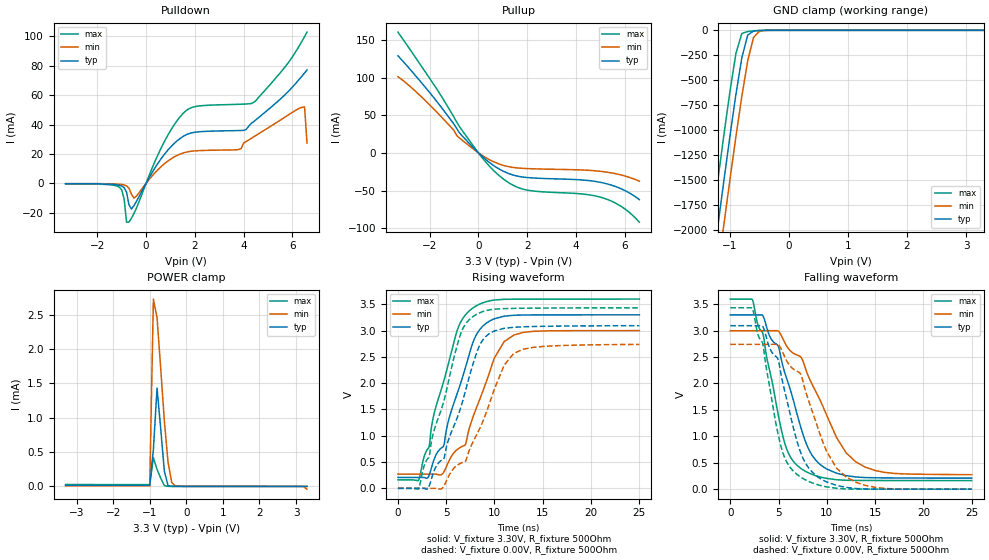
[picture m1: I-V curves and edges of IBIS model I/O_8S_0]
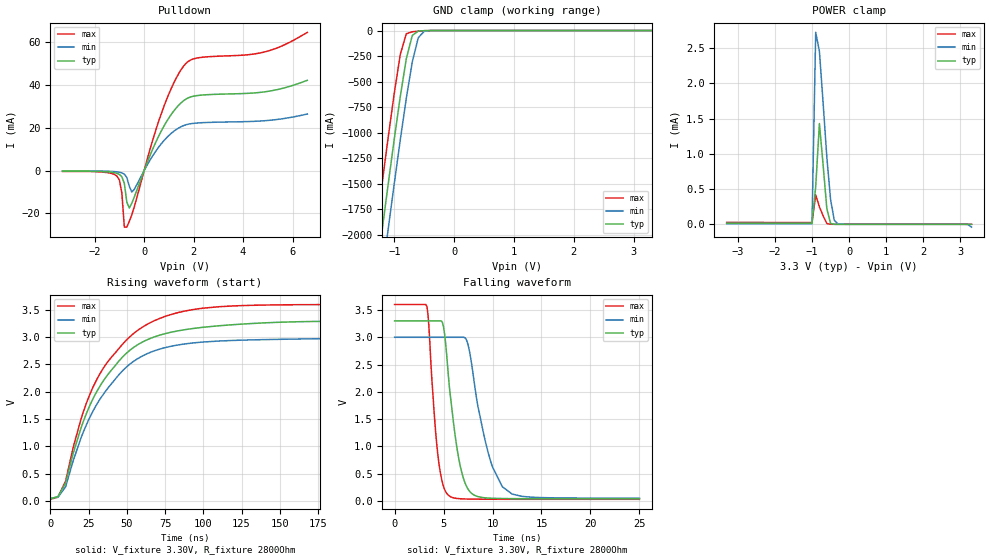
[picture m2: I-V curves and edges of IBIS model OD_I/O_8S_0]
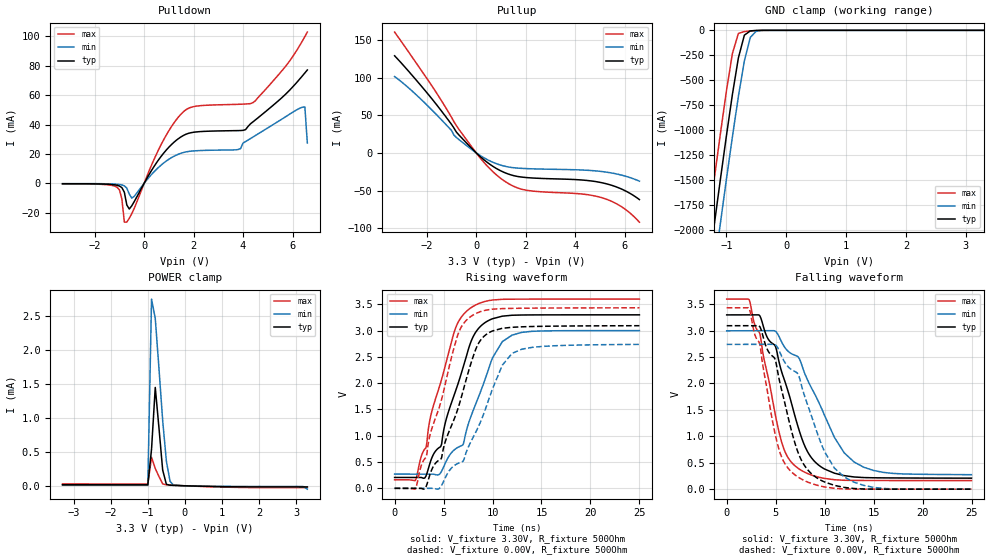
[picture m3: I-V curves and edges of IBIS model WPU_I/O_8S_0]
[IBIS Ver]   3.2
[File Name]   lm3s2651_lqfp_v0p1.ibs
[File Rev]   0.1
[Date]   02/19/2010
[Source]   From silicon level SPICE simulations at Texas Instruments
[Notes]   Initial Release of IBIS model
   LM3S2651, Revision A2, 100 LQFP
[Disclaimer] Texas Instruments Confidential - Advance Product Information
   < Software License Agreement >
  Texas Instruments (TI) is supplying this software for use solely and
  exclusively on TI's Stellaris Family of microcontroller products.
  The software is owned by TI and/or its suppliers, and is protected under
  applicable copyright laws.  All rights are reserved.  Any use in violation
  of the foregoing restrictions may subject the user to criminal sanctions
  under applicable laws, as well as to civil liability for the breach of the
  terms and conditions of this license.
  THIS SOFTWARE IS PROVIDED "AS IS".  NO WARRANTIES, WHETHER EXPRESS, IMPLIED
  OR STATUTORY, INCLUDING, BUT NOT LIMITED TO, IMPLIED WARRANTIES OF
  MERCHANTABILITY AND FITNESS FOR A PARTICULAR PURPOSE APPLY TO THIS SOFTWARE.
  LMI SHALL NOT, IN ANY CIRCUMSTANCES, BE LIABLE FOR SPECIAL, INCIDENTAL, OR
  CONSEQUENTIAL DAMAGES, FOR ANY REASON WHATSOEVER.
[Copyright]   Copyright (c) 2010 Texas Instruments.  All rights reserved.
[Component]   LM3S2651 100LQFP
[Manufacturer]  Texas Instruments
[Package]
| 100-pin LQFP
| variable   typ   min   max
R_pkg   125.000m   98.000m   152.000m
L_pkg   7.745nH   6.720nH   8.770nH
C_pkg   0.745pF   0.660pF   0.830pF
[Pin]  signal_name   model_name
   1   ADC0   NC
   2   ADC1   NC
   3   VDDA   POWER
   4   GNDA   GND
   5   ADC2   NC
   6   ADC3   NC
   7   LDO   POWER
   8   VDD   POWER
   9   GND   GND
  10   PD0_CAN0Rx   ProgBuff1
  11   PD1_CAN0Tx   ProgBuff1
  12   PD2_U1Rx   ProgBuff1
  13   PD3_U1Tx   ProgBuff1
  14   VDD25   POWER
  15   GND   GND
  16   PG3   ProgBuff2
  17   PG2   ProgBuff2
  18   PG1_U2Tx   ProgBuff1
  19   PG0_U2Rx   ProgBuff1
  20   VDD   POWER
  21   GND   GND
  22   NC   NC
  23   PC6_CCP3   ProgBuff1
  24   PC5_C0o   ProgBuff1
  25   PC4   ProgBuff1
  26   PA0_U0Rx   ProgBuff1
  27   PA1_U0Tx   ProgBuff1
  28   PA2_SSI0Clk   ProgBuff1
  29   PA3_SSI0Fss   ProgBuff1
  30   PA4_SSI0Rx   ProgBuff1
  31   PA5_SSI0Tx   ProgBuff1
  32   VDD   POWER
  33   GND   GND
  34   PA6_CCP1   ProgBuff1
  35   PA7_CCP4   ProgBuff1
  36   PG7   ProgBuff2
  37   PG6   ProgBuff2
  38   VDD25   POWER
  39   GND   GND
  40   PG5   ProgBuff2
  41   PG4   ProgBuff2
  42   PF7   ProgBuff2
  43   PF6   ProgBuff2
  44   VDD   POWER
  45   GND   GND
  46   PF5   ProgBuff2
  47   PF0_PWM0   ProgBuff1
  48   OSC0   NC
  49   OSC1   NC
  50   WAKE   NC
  51   HIB   NC
  52   XOSC0   NC
  53   XOSC1   NC
  54   GND   GND
  55   VBAT   POWER
  56   VDD   POWER
  57   GND   GND
  58   PF4   ProgBuff1
  59   PF3   ProgBuff1
  60   PF2   ProgBuff1
  61   PF1_PWM1   ProgBuff1
  62   VDD25   POWER
  63   GND   GND
  64   RST   NC
  65   CMOD0   NC
  66   PB0_CCP0   ProgBuff1
  67   PB1_CCP2   ProgBuff1
  68   VDD   POWER
  69   GND   GND
  70   PB2_I2C0SCL   ProgBuff1
  71   PB3_I2C0SDA   ProgBuff1
  72   PE0_SSI1Clk   ProgBuff1
  73   PE1_SSI1Fss   ProgBuff1
  74   PE2_SSI1Rx   ProgBuff1
  75   PE3_SSI1Tx   ProgBuff1
  76   CMOD1   NC
  77   PC3_TDO_SWO   ProgBuff1
  78   PC2_TDI   ProgBuff1
  79   PC1_TMS_SWDIO   ProgBuff1
  80   PC0_TCK_SWCLK   ProgBuff1
  81   VDD   POWER
  82   GND   GND
  83   NC   NC
  84   NC   NC
  85   PH1_PWM3   ProgBuff2
  86   PH0_PWM2   ProgBuff2
  87   GND   GND
  88   VDD25   POWER
  89   PB7_TRST   ProgBuff1
  90   PB6   ProgBuff1
  91   PB5_CCP5   ProgBuff1
  92   PB4   ProgBuff1
  93   VDD   POWER
  94   GND   GND
  95   PD4   ProgBuff0
  96   PD5   ProgBuff0
  97   GNDA   GND
  98   VDDA   POWER
  99   PD6_Fault   ProgBuff0
 100   PD7   ProgBuff0
[Model Selector]   ProgBuff0
I/O_2_0   2 mA buffer without slew rate control
I/O_4_0   4 mA buffer without slew rate control
I/O_8_0   8 mA buffer without slew rate control
I/O_8S_0   8 mA buffer with slew rate control
OD_I/O_2_0   open-drain 2 mA buffer without slew rate control
OD_I/O_4_0   open-drain 4 mA buffer without slew rate control
OD_I/O_8_0   open-drain 8 mA buffer without slew rate control
OD_I/O_8S_0   open-drain 8 mA buffer with slew rate control
WPU_I/O_2_0   weak pullup 2 mA buffer without slew rate control
WPU_I/O_4_0   weak pullup 4 mA buffer without slew rate control
WPU_I/O_8_0   weak pullup 8 mA buffer without slew rate control
WPU_I/O_8S_0   weak pullup 8 mA buffer with slew rate control
WPD_I/O_2_0   weak pulldown 2 mA buffer without slew rate control
WPD_I/O_4_0   weak pulldown 4 mA buffer without slew rate control
WPD_I/O_8_0   weak pulldown 8 mA buffer without slew rate control
WPD_I/O_8S_0   weak pulldown 8 mA buffer with slew rate control
[Model Selector]   ProgBuff1
I/O_2_1   2 mA buffer without slew rate control
I/O_4_1   4 mA buffer without slew rate control
I/O_8_1   8 mA buffer without slew rate control
I/O_8S_1   8 mA buffer with slew rate control
OD_I/O_2_1   open-drain 2 mA buffer without slew rate control
OD_I/O_4_1   open-drain 4 mA buffer without slew rate control
OD_I/O_8_1   open-drain 8 mA buffer without slew rate control
OD_I/O_8S_1   open-drain 8 mA buffer with slew rate control
WPU_I/O_2_1   weak pullup 2 mA buffer without slew rate control
WPU_I/O_4_1   weak pullup 4 mA buffer without slew rate control
WPU_I/O_8_1   weak pullup 8 mA buffer without slew rate control
WPU_I/O_8S_1   weak pullup 8 mA buffer with slew rate control
WPD_I/O_2_1   weak pulldown 2 mA buffer without slew rate control
WPD_I/O_4_1   weak pulldown 4 mA buffer without slew rate control
WPD_I/O_8_1   weak pulldown 8 mA buffer without slew rate control
WPD_I/O_8S_1   weak pulldown 8 mA buffer with slew rate control
[Model Selector]   ProgBuff2
I/O_2_2   2 mA buffer without slew rate control
I/O_4_2   4 mA buffer without slew rate control
I/O_8_2   8 mA buffer without slew rate control
I/O_8S_2   8 mA buffer with slew rate control
OD_I/O_2_2   open-drain 2 mA buffer without slew rate control
OD_I/O_4_2   open-drain 4 mA buffer without slew rate control
OD_I/O_8_2   open-drain 8 mA buffer without slew rate control
OD_I/O_8S_2   open-drain 8 mA buffer with slew rate control
WPU_I/O_2_2   weak pullup 2 mA buffer without slew rate control
WPU_I/O_4_2   weak pullup 4 mA buffer without slew rate control
WPU_I/O_8_2   weak pullup 8 mA buffer without slew rate control
WPU_I/O_8S_2   weak pullup 8 mA buffer with slew rate control
WPD_I/O_2_2   weak pulldown 2 mA buffer without slew rate control
WPD_I/O_4_2   weak pulldown 4 mA buffer without slew rate control
WPD_I/O_8_2   weak pulldown 8 mA buffer without slew rate control
WPD_I/O_8S_2   weak pulldown 8 mA buffer with slew rate control
| Models and submodels in the file (48): I/O_2_0 (I/O), I/O_4_0 (I/O), I/O_8_0 (I/O), I/O_8S_0 (I/O), OD_I/O_2_0 (I/O_open_drain), OD_I/O_4_0 (I/O_open_drain), OD_I/O_8_0 (I/O_open_drain), OD_I/O_8S_0 (I/O_open_drain), WPU_I/O_2_0 (I/O), WPU_I/O_4_0 (I/O), WPU_I/O_8_0 (I/O), WPU_I/O_8S_0 (I/O), WPD_I/O_2_0 (I/O), WPD_I/O_4_0 (I/O), WPD_I/O_8_0 (I/O), WPD_I/O_8S_0 (I/O), I/O_2_1 (I/O), I/O_4_1 (I/O), I/O_8_1 (I/O), I/O_8S_1 (I/O), OD_I/O_2_1 (I/O_open_drain), OD_I/O_4_1 (I/O_open_drain), OD_I/O_8_1 (I/O_open_drain), OD_I/O_8S_1 (I/O_open_drain), WPU_I/O_2_1 (I/O), WPU_I/O_4_1 (I/O), WPU_I/O_8_1 (I/O), WPU_I/O_8S_1 (I/O), WPD_I/O_2_1 (I/O), WPD_I/O_4_1 (I/O), WPD_I/O_8_1 (I/O), WPD_I/O_8S_1 (I/O), I/O_2_2 (I/O), I/O_4_2 (I/O), I/O_8_2 (I/O), I/O_8S_2 (I/O), OD_I/O_2_2 (I/O_open_drain), OD_I/O_4_2 (I/O_open_drain), OD_I/O_8_2 (I/O_open_drain), OD_I/O_8S_2 (I/O_open_drain), WPU_I/O_2_2 (I/O), WPU_I/O_4_2 (I/O), WPU_I/O_8_2 (I/O), WPU_I/O_8S_2 (I/O), WPD_I/O_2_2 (I/O), WPD_I/O_4_2 (I/O), WPD_I/O_8_2 (I/O), WPD_I/O_8S_2 (I/O)
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[Model]   I/O_8S_0
Model_type   I/O
Vinl = 1.26
Vinh = 2.04
Vmeas = 1.65
| variable   typ   min   max
C_comp   9.739pF   9.739pF   9.739pF
[Model Spec]
Vinh+   1.91   1.78   2.04
Vinh-   1.90   1.76   2.03
Vinl+   1.40   1.27   1.54
Vinl-   1.39   1.26   1.53
| variable   typ   min   max
[Temperature Range]  25   85   -40
[Voltage Range]   3.3V   3.0V   3.6V
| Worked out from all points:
|   slope of the pulldown table from 0 to 0.495 V, typ, clamps not added: 35.8 ohm
|   slope of the pullup table from 0 to 0.495 V, typ, clamps not added: 35.8 ohm
|   GND clamp passes 1 mA (typ) near -0.48 V on its own axis
|   POWER clamp passes 1 mA (typ) near -0.73 V on its own axis
|   falling waveform, V_fixture 3.30V, R_fixture 500Ohm: 20-80 % time 2.93ns typ, 4.09ns min, 2.25ns max; typ from 3.3 V to 0.208 V
|   rising waveform, V_fixture 3.30V, R_fixture 500Ohm: 20-80 % time 2.83ns typ, 3.04ns min, 2.71ns max; typ from 0.208 V to 3.3 V
|   falling waveform, V_fixture 0.00V, R_fixture 500Ohm: 20-80 % time 2.55ns typ, 3.29ns min, 2.08ns max; typ from 3.09 V to 0 V
|   rising waveform, V_fixture 0.00V, R_fixture 500Ohm: 20-80 % time 3.13ns typ, 3.58ns min, 2.86ns max; typ from 0 V to 3.09 V
[Pulldown]
|  Voltage   I(typ)   I(min)   I(max)
-3.3V     -256.6uA   -145.6uA   -364.5uA
-1.1V     -1.273mA   -587.5uA   -2.567mA
-900mV    -2.885mA   -1.061mA   -10.54mA
-800mV    -5.993mA   -1.67mA    -26.39mA
-700mV    -14.71mA   -3.215mA   -26.33mA
-500mV    -15.26mA   -10mA      -20.66mA
600mV     16.36mA    11.13mA    23.41mA
1.5V      31.68mA    20.52mA    47.2mA
3.8V      35.88mA    22.99mA    53.74mA
4.4V      41.81mA    31.48mA    54.89mA
6.5V      75.06mA    51.95mA    99.78mA
6.6V      77.08mA    27.42mA    102.8mA
[Pullup]
|  Voltage   I(typ)   I(min)   I(max)
-3.3V     128.9mA    101.3mA    160.4mA
-2V       80.13mA    63.77mA    99.04mA
-1V       37.9mA     29.83mA    47.32mA
-700mV    23.81mA    17.7mA     31.28mA
300mV     -8.845mA   -6.303mA   -12.15mA
1V        -23.99mA   -16.37mA   -34.1mA
1.5V      -30.13mA   -19.7mA    -44.22mA
2V        -32.73mA   -20.87mA   -49.46mA
4.3V      -36.12mA   -22.8mA    -54.75mA
5.1V      -39.81mA   -24.88mA   -59.77mA
5.9V      -48.4mA    -29.75mA   -72.06mA
6.6V      -62.06mA   -37.61mA   -92.08mA
[GND Clamp]
|  Voltage   I(typ)   I(min)   I(max)
-3.3V     -11.72A    -12.12A    -11.3A
-1.4V     -2.845A    -3.285A    -2.387A
-1.3V     -2.39A     -2.831A    -1.93A
-1.2V     -1.938A    -2.38A     -1.478A
-1.1V     -1.494A    -1.934A    -1.036A
-1V       -1.059A    -1.496A    -610.6mA
-900mV    -645mA     -1.069A    -232.9mA
-800mV    -277.1mA   -664.4mA   -31.59mA
-700mV    -48.56mA   -306.6mA   -12.09mA
-600mV    -5.558mA   -70.2mA    -6.272mA
-500mV    -1.167mA   -7.88mA    -2.167mA
3.3V      2.282nA    3.101uA    451.3pA
[POWER Clamp]
|  Voltage   I(typ)   I(min)   I(max)
-3.3V     15.18uA    8.315uA    27.48uA
-1V       14.14uA    7.74uA     25.63uA
-900mV    536uA      2.726mA    416.7uA
-800mV    1.43mA     2.454mA    247.6uA
-700mV    840.7uA    1.719mA    119.9uA
-600mV    221.2uA    951.5uA    11.58uA
-500mV    12.35uA    355.6uA    955.3nA
-400mV    305.2nA    58.59uA    44.3nA
-300mV    9.515nA    3.101uA    1.472nA
3.1V      1.302nA    -112.7nA   143.5pA
3.2V      1.207nA    -2.287uA   131.7pA
3.3V      -104.8pA   -40.34uA   119.2pA
[Ramp]
| variable   typ   min   max
dV/dt_f   1.85/2.93n   1.63/4.09n   2.06/2.25n
dV/dt_r   1.85/3.13n   1.64/3.58n   2.06/2.86n
R_load = 500Ohm
[Falling Waveform]
V_fixture = 3.30V
V_fixture_min = 3.00V
V_fixture_max = 3.60V
R_fixture = 500Ohm
|   Time   V(typ)   V(min)   V(max)
0s        3.298V     2.996V     3.597V
2.3ns     3.298V     2.998V     3.585V
3.4ns     3.276V     2.998V     2.936V
5ns       2.692V     2.987V     1.378V
5.6ns     2.229V     2.79V      898.3mV
7.2ns     1.235V     2.517V     407.7mV
9.1ns     502.1mV    1.761V     241.2mV
11ns      302.3mV    979.8mV    178.8mV
13ns      231mV      515.9mV    165.4mV
25ns      208.4mV    274.1mV    162.4mV
[Rising Waveform]
V_fixture = 3.30V
V_fixture_min = 3.00V
V_fixture_max = 3.60V
R_fixture = 500Ohm
|   Time   V(typ)   V(min)   V(max)
0s        207.7mV    271.2mV    162.2mV
2.1ns     207.5mV    270.5mV    146.6mV
3.2ns     232.7mV    270.2mV    771.4mV
4.8ns     840.9mV    326.1mV    2.073V
6.1ns     1.783V     732.4mV    2.98V
7ns       2.303V     833.1mV    3.299V
7.7ns     2.739V     1.319V     3.42V
10ns      3.225V     2.483V     3.58V
12ns      3.291V     2.913V     3.596V
25ns      3.299V     2.999V     3.598V
[Falling Waveform]
V_fixture = 0.00V
V_fixture_min = 0.00V
V_fixture_max = 0.00V
R_fixture = 500Ohm
|   Time   V(typ)   V(min)   V(max)
0s        3.093V     2.739V     3.433V
2.3ns     3.093V     2.74V      3.421V
3.4ns     3.071V     2.74V      2.73V
4.9ns     2.477V     2.739V     1.087V
5.3ns     2.13V      2.643V     778.7mV
7ns       852.9mV    2.223V     266.6mV
8.1ns     406.7mV    1.685V     148.2mV
10ns      135.5mV    708.4mV    42.72mV
12ns      33.41mV    230.5mV    3.849mV
25ns      39.44uV    90.62uV    23.66uV
[Rising Waveform]
V_fixture = 0.00V
V_fixture_min = 0.00V
V_fixture_max = 0.00V
R_fixture = 500Ohm
|   Time   V(typ)   V(min)   V(max)
0s        402.7uV    2.355mV    175.9uV
2.1ns     186.9uV    995.9uV    -14.86mV
3.1ns     -4.815mV   567.3uV    569mV
4.6ns     543.7mV    4.108mV    1.563V
6.4ns     1.478V     468.1mV    2.886V
7.7ns     2.319V     853mV      3.256V
9.1ns     2.885V     1.418V     3.377V
11ns      3.043V     2.342V     3.417V
12ns      3.062V     2.567V     3.421V
25ns      3.092V     2.736V     3.432V
[Model]   OD_I/O_8S_0
Model_type   I/O_open_drain
Polarity   Inverting
Vinl = 1.26
Vinh = 2.04
Vmeas = 1.65
Rref = 2800
Vref = 3.3
| variable   typ   min   max
C_comp   9.739pF   9.739pF   9.739pF
[Model Spec]
Vinh+   1.91   1.78   2.04
Vinh-   1.90   1.76   2.03
Vinl+   1.40   1.27   1.54
Vinl-   1.39   1.26   1.53
| variable   typ   min   max
[Temperature Range]  25   85   -40
[Voltage Range]   3.3V   3.0V   3.6V
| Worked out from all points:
|   slope of the pulldown table from 0 to 0.495 V, typ, clamps not added: 35.8 ohm
|   GND clamp passes 1 mA (typ) near -0.48 V on its own axis
|   POWER clamp passes 1 mA (typ) near -0.73 V on its own axis
|   falling waveform, V_fixture 3.30V, R_fixture 2800Ohm: 20-80 % time 1.32ns typ, 2.02ns min, 884ps max; typ from 3.3 V to 0.038 V
|   rising waveform, V_fixture 3.30V, R_fixture 2800Ohm: 20-80 % time 34.2ns typ, 34ns min, 34.6ns max; typ from 0.038 V to 3.3 V
[Pulldown]
|  Voltage   I(typ)   I(min)   I(max)
-3.3V     -256.6uA   -145.6uA   -364.5uA
-1.1V     -1.273mA   -587.5uA   -2.567mA
-900mV    -2.885mA   -1.061mA   -10.54mA
-800mV    -5.993mA   -1.67mA    -26.39mA
-700mV    -14.71mA   -3.215mA   -26.33mA
-600mV    -17.43mA   -7.321mA   -23.73mA
-500mV    -15.26mA   -10mA      -20.66mA
700mV     18.62mA    12.61mA    26.75mA
1.2V      27.84mA    18.36mA    40.91mA
1.7V      33.44mA    21.41mA    50.13mA
4.9V      36.8mA     23.3mA     55.47mA
6.6V      42.15mA    26.42mA    64.53mA
[GND Clamp]
|  Voltage   I(typ)   I(min)   I(max)
-3.3V     -11.72A    -12.12A    -11.3A
-1.4V     -2.845A    -3.285A    -2.387A
-1.3V     -2.39A     -2.831A    -1.93A
-1.2V     -1.938A    -2.38A     -1.478A
-1.1V     -1.494A    -1.934A    -1.036A
-1V       -1.059A    -1.496A    -610.6mA
-900mV    -645mA     -1.069A    -232.9mA
-800mV    -277.1mA   -664.4mA   -31.59mA
-700mV    -48.56mA   -306.6mA   -12.09mA
-600mV    -5.558mA   -70.2mA    -6.272mA
-500mV    -1.167mA   -7.88mA    -2.167mA
3.3V      2.282nA    3.101uA    451.3pA
[POWER Clamp]
|  Voltage   I(typ)   I(min)   I(max)
-3.3V     15.18uA    8.315uA    27.48uA
-1V       14.14uA    7.74uA     25.63uA
-900mV    536uA      2.726mA    416.7uA
-800mV    1.43mA     2.454mA    247.6uA
-700mV    840.7uA    1.719mA    119.9uA
-600mV    221.2uA    951.5uA    11.58uA
-500mV    12.35uA    355.6uA    955.3nA
-400mV    305.2nA    58.59uA    44.3nA
-300mV    9.515nA    3.101uA    1.472nA
3.1V      1.302nA    -112.7nA   143.5pA
3.2V      1.207nA    -2.287uA   131.7pA
3.3V      -104.8pA   -40.34uA   119.2pA
[Ramp]
| variable   typ   min   max
dV/dt_f   1.96/1.32n   1.77/2.02n   2.14/0.88n
dV/dt_r   1.96/34.24n   1.77/34.01n   2.14/34.63n
R_load = 2800Ohm
[Falling Waveform]
V_fixture = 3.30V
V_fixture_min = 3.00V
V_fixture_max = 3.60V
R_fixture = 2800Ohm
|   Time   V(typ)   V(min)   V(max)
0s        3.3V       2.999V     3.6V
3.3ns     3.3V       2.999V     3.564V
4.4ns     3.3V       2.999V     872.1mV
5ns       3.186V     2.999V     262.6mV
5.5ns     2.279V     2.999V     103.6mV
6.4ns     934mV      2.999V     44.88mV
7.3ns     283.8mV    2.965V     35.58mV
9.4ns     54.75mV    993.7mV    31.53mV
11ns      44.17mV    261mV      30.69mV
25ns      37.97mV    50.43mV    29.46mV
[Rising Waveform]
V_fixture = 3.30V
V_fixture_min = 3.00V
V_fixture_max = 3.60V
R_fixture = 2800Ohm
|   Time   V(typ)   V(min)   V(max)
0s        38.08mV    50.7mV     29.48mV
5ns       80.81mV    66.81mV    69.32mV
10ns      324.3mV    257.9mV    361.8mV
20ns      1.329V     1.148V     1.491V
32ns      2.082V     1.844V     2.308V
49ns      2.686V     2.433V     2.925V
65ns      2.973V     2.718V     3.261V
85ns      3.124V     2.865V     3.461V
110ns     3.209V     2.93V      3.558V
250ns     3.298V     2.994V     3.599V
[Model]   WPU_I/O_8S_0
Model_type   I/O
Vinl = 1.26
Vinh = 2.04
Vmeas = 1.65
| variable   typ   min   max
C_comp   9.739pF   9.739pF   9.739pF
[Model Spec]
Vinh+   1.91   1.78   2.04
Vinh-   1.90   1.76   2.03
Vinl+   1.40   1.27   1.54
Vinl-   1.39   1.26   1.53
| variable   typ   min   max
[Temperature Range]  25   85   -40
[Voltage Range]   3.3V   3.0V   3.6V
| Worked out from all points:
|   slope of the pulldown table from 0 to 0.495 V, typ, clamps not added: 35.8 ohm
|   slope of the pullup table from 0 to 0.495 V, typ, clamps not added: 35.8 ohm
|   GND clamp passes 1 mA (typ) near -0.48 V on its own axis
|   POWER clamp passes 1 mA (typ) near -0.73 V on its own axis
|   falling waveform, V_fixture 3.30V, R_fixture 500Ohm: 20-80 % time 2.93ns typ, 4.09ns min, 2.25ns max; typ from 3.3 V to 0.208 V
|   rising waveform, V_fixture 3.30V, R_fixture 500Ohm: 20-80 % time 2.83ns typ, 3.04ns min, 2.71ns max; typ from 0.208 V to 3.3 V
|   falling waveform, V_fixture 0.00V, R_fixture 500Ohm: 20-80 % time 2.55ns typ, 3.29ns min, 2.08ns max; typ from 3.09 V to 0 V
|   rising waveform, V_fixture 0.00V, R_fixture 500Ohm: 20-80 % time 3.13ns typ, 3.58ns min, 2.86ns max; typ from 0 V to 3.09 V
[Pulldown]
|  Voltage   I(typ)   I(min)   I(max)
-3.3V     -256.4uA   -145.5uA   -364.3uA
-1.1V     -1.272mA   -586.9uA   -2.565mA
-900mV    -2.884mA   -1.06mA    -10.53mA
-800mV    -5.991mA   -1.669mA   -26.38mA
-700mV    -14.71mA   -3.213mA   -26.31mA
-500mV    -15.24mA   -9.997mA   -20.64mA
600mV     16.38mA    11.14mA    23.43mA
1.5V      31.7mA     20.53mA    47.23mA
3.8V      35.88mA    22.99mA    53.74mA
4.4V      41.81mA    31.48mA    54.88mA
6.5V      75.06mA    51.95mA    99.78mA
6.6V      77.08mA    27.42mA    102.8mA
[Pullup]
|  Voltage   I(typ)   I(min)   I(max)
-3.3V     128.9mA    101.3mA    160.4mA
-2V       80.13mA    63.77mA    99.04mA
-1V       37.9mA     29.83mA    47.32mA
-700mV    23.8mA     17.69mA    31.27mA
300mV     -8.84mA    -6.3mA     -12.15mA
1V        -23.98mA   -16.37mA   -34.08mA
1.5V      -30.12mA   -19.69mA   -44.19mA
2V        -32.71mA   -20.86mA   -49.43mA
4.3V      -36.12mA   -22.8mA    -54.73mA
5.1V      -39.81mA   -24.88mA   -59.77mA
5.9V      -48.4mA    -29.75mA   -72.06mA
6.6V      -62.06mA   -37.61mA   -92.08mA
[GND Clamp]
|  Voltage   I(typ)   I(min)   I(max)
-3.3V     -11.72A    -12.12A    -11.3A
-1.4V     -2.845A    -3.285A    -2.387A
-1.3V     -2.39A     -2.831A    -1.93A
-1.2V     -1.938A    -2.38A     -1.478A
-1.1V     -1.494A    -1.934A    -1.036A
-1V       -1.059A    -1.496A    -610.6mA
-900mV    -645mA     -1.069A    -232.9mA
-800mV    -277.1mA   -664.4mA   -31.6mA
-700mV    -48.56mA   -306.6mA   -12.11mA
-600mV    -5.565mA   -70.2mA    -6.295mA
-500mV    -1.181mA   -7.883mA   -2.191mA
3.3V      2.282nA    6.919uA    -6.845uA
[POWER Clamp]
|  Voltage   I(typ)   I(min)   I(max)
-3.3V     15.18uA    8.315uA    27.48uA
-1V       14.14uA    7.74uA     25.63uA
-900mV    539.2uA    2.746mA    419.4uA
-800mV    1.446mA    2.463mA    255uA
-700mV    851uA      1.726mA    135.8uA
-600mV    231.3uA    957.3uA    27.23uA
-500mV    21.69uA    361.2uA    14.14uA
-400mV    7.764uA    63.51uA    10.49uA
-300mV    5.5uA      6.919uA    7.727uA
3.1V      -16.64uA   -9.947uA   -27.43uA
3.2V      -16.65uA   -12.11uA   -27.44uA
3.3V      -16.65uA   -49.87uA   -27.45uA
[Ramp]
| variable   typ   min   max
dV/dt_f   1.85/2.93n   1.63/4.09n   2.06/2.25n
dV/dt_r   1.85/3.13n   1.64/3.58n   2.06/2.86n
R_load = 500Ohm
[Falling Waveform]
V_fixture = 3.30V
V_fixture_min = 3.00V
V_fixture_max = 3.60V
R_fixture = 500Ohm
|   Time   V(typ)   V(min)   V(max)
0s        3.298V     2.996V     3.597V
2.3ns     3.298V     2.998V     3.585V
3.4ns     3.276V     2.998V     2.936V
5ns       2.692V     2.987V     1.378V
5.6ns     2.229V     2.79V      898.3mV
7.2ns     1.235V     2.517V     407.7mV
9.1ns     502.1mV    1.761V     241.2mV
11ns      302.3mV    979.8mV    178.8mV
13ns      231mV      515.9mV    165.4mV
25ns      208.4mV    274.1mV    162.4mV
[Rising Waveform]
V_fixture = 3.30V
V_fixture_min = 3.00V
V_fixture_max = 3.60V
R_fixture = 500Ohm
|   Time   V(typ)   V(min)   V(max)
0s        207.7mV    271.2mV    162.2mV
2.1ns     207.5mV    270.5mV    146.6mV
3.2ns     232.7mV    270.2mV    771.4mV
4.8ns     840.9mV    326.1mV    2.073V
6.1ns     1.783V     732.4mV    2.98V
7ns       2.303V     833.1mV    3.299V
7.7ns     2.739V     1.319V     3.42V
10ns      3.225V     2.483V     3.58V
12ns      3.291V     2.913V     3.596V
25ns      3.299V     2.999V     3.598V
[Falling Waveform]
V_fixture = 0.00V
V_fixture_min = 0.00V
V_fixture_max = 0.00V
R_fixture = 500Ohm
|   Time   V(typ)   V(min)   V(max)
0s        3.093V     2.739V     3.433V
2.3ns     3.093V     2.74V      3.421V
3.4ns     3.071V     2.74V      2.73V
4.9ns     2.477V     2.739V     1.087V
5.3ns     2.13V      2.643V     778.7mV
7ns       852.9mV    2.223V     266.6mV
8.1ns     406.7mV    1.685V     148.2mV
10ns      135.5mV    708.4mV    42.72mV
12ns      33.41mV    230.5mV    3.849mV
25ns      39.44uV    90.62uV    23.66uV
[Rising Waveform]
V_fixture = 0.00V
V_fixture_min = 0.00V
V_fixture_max = 0.00V
R_fixture = 500Ohm
|   Time   V(typ)   V(min)   V(max)
0s        401.3uV    2.355mV    176.7uV
2.1ns     186.9uV    996.5uV    -14.86mV
3.1ns     -4.815mV   567.6uV    569mV
4.6ns     543.7mV    4.107mV    1.563V
6.4ns     1.478V     468.1mV    2.886V
7.7ns     2.319V     853mV      3.256V
9.1ns     2.885V     1.418V     3.377V
11ns      3.043V     2.342V     3.417V
12ns      3.062V     2.567V     3.421V
25ns      3.092V     2.736V     3.432V
